(* Logix 5000 Rung export; software revision 16.04 *)

MODULES
   Local : vendor None type None code None
   EGD : vendor None type None code None
END_MODULES

TYPE SNTPStat :   // Simple Network Time Protocol statistics.
STRUCT
   ValidTime : INT;   // SNTP valid time
   ReqCnt : INT;   // SNTP request count
   RespCnt : INT;   // SNTP response count
   CompCnt : INT;   // SNTP computation count
   SetCnt : INT;   // SNTP set count
   TimeoutErrCnt : INT;   // SNTP timeout error count
   SecLSW : INT;   // SNTP seconds (LSW)
   SecMSW : INT;   // SNTP seconds (MSW)
   micSecLSW : INT;   // SNTP microseconds (LSW)
   micSecMSW : INT;   // SNTP microseconds (MSW)
   Sec : DINT;   // SNTP seconds
   micSec : DINT;   // SNTP microseconds
END_STRUCT
END_TYPE

TYPE InStat :   // This status data is returned on each read block and can be used to detect proper module operation.
STRUCT
   PassCnt : INT;   // Program cycle/scan counter
   BlkCntr : BlkStat;   // Block counter statistics
   SNTP : SNTPStat;   // Simple Network Time Protocol statistics
END_STRUCT
END_TYPE

TYPE EGDCONTROL :   // Stores control registers used by the processor to request special tasks from the module.
STRUCT
   ColdBoot : BOOL;   // Total SW/HW module reset
   WarmBoot : BOOL;   // Configuration parameter reset
   CPmessage : CPStat[17];   // CP message status
   CPmessReq : BOOL;   // Initiates Block 2000. C/P Messages
   CPmessReqQty : INT;   // Quantity of Consumer/Producer Message
   CPindxFirst : INT;   // Index of the First Consumer/Producer Message
   CPmessResQty : INT;   // Quantity of Consumer/Producer Message from Module
   CPindxResFirst : INT;   // Index of the First Consumer/Producer Message from Module
   CPwordsQty : INT;   // Calculated words Qty CP messages x 14.
   PortErrors : PortErrors;   // This encapsulates all port error statistics.
END_STRUCT
END_TYPE

TYPE BlkStat :   // Block Transfer Statistics
STRUCT
   Write : INT;   // Total number of write block transfers. Block Write counter.
   Read : INT;   // Total number of read block transfers. Block Read counter.
   Parse : INT;   // Total number of blocks parsed. Block Parse counter.
   Error : INT;   // Total number of block transfer errors. Block Error Counter.
END_STRUCT
END_TYPE

TYPE EGDMODULEDEF :   // MVI56-EGD module definitions.
STRUCT
   DATA : EGDDATA;   // Stores the database (read and write) values.
   CONTROL : EGDCONTROL;   // Stores control registers used by the processor to request special tasks from the module.
   STATUS : EGDSTATUS;   // Stores status registers.
   UTIL : EGDUTIL;   // Stores tags that are used by the ladder logic for internal processing.
END_STRUCT
END_TYPE

TYPE Blk9250Stat :   // Block 9250 Response Block general status
STRUCT
   BlkWriteIDreq : INT;   // Block Write ID Requested
   PassCnt : INT;   // Program Scan Counter
   ProdCodeByte0 : SINT;   // Product code byte 0 of 0 & 1
   ProdCodeByte1 : SINT;   // Product code byte 1 of 0 & 1
   ProdCodeByte2 : SINT;   // Product code byte 2 of 2 & 3
   ProdCodeByte3 : SINT;   // Product code byte 3 of 2 & 3
   RevByte0 : SINT;   // Revision byte 0 of 0 & 1
   RevByte1 : SINT;   // Revision byte 1 of 0 & 1
   RevByte2 : SINT;   // Revision byte 2 of 2 & 3
   RevByte3 : SINT;   // Revision byte 3 of 2 & 3
   OpByte0 : SINT;   // Op byte 0 of 0 & 1
   OpByte1 : SINT;   // Op byte 1 of 0 & 1
   OpByte2 : SINT;   // Op byte 2 of 2 & 3
   OpByte3 : SINT;   // Op byte 3 of 2 & 3
   RunByte0 : SINT;   // Run byte 0 of 0 & 1
   RunByte1 : SINT;   // Run byte 1 of 0 & 1
   RunByte2 : SINT;   // Run byte 2 of 2 & 3
   RunByte3 : SINT;   // Run byte 3 of 2 & 3
   BlkXferStat : BlkStat;   // Block transfer statistics
   ProductCodeName : DINT;   // Product code name
   RevisionLevel : DINT;   // Firmware revision level
   OpSysRevision : DINT;   // Operating system revision level
   RunNumber : DINT;   // Run number
END_STRUCT
END_TYPE

TYPE CPStat :   // Block 2000 Each Conmsumer/Producer Status Data
STRUCT
   Status : INT;   // Status (0=invalid, 1=producing/healthy, 2=pending/unhealthy)
   StatBit : INT;   // Status bit mapped (bit 0=error or invalid, bit 1=not time synchronized, bits 2 to 15 reserved)
   CPnumTimesLSW : INT;   // Number of times C/P (LSW)
   CPnumTimesMSW : INT;   // Number of times C/P (MSW)
   MissCntLSW : INT;   // Missed count (LSW)
   MissCntMSW : INT;   // Missed count (MSW)
   RfrshCntErrLSW : INT;   // Refresh count error (LSW)
   RfrshCntErrMSW : INT;   // Refresh count error (MSW)
   InvErrBit : INT;   // Invalid error bit set by producer
   TimeSyncErr : INT;   // Time sync error set by producer
   ShrtMEsgErr : INT;   // Short message error in exchange
   LngMEsgErr : INT;   // Long message error in exchange
   PrtclPVN : INT;   // Protocol PVN not set to 1
   CnfgSig : INT;   // Configuration signature not set correctly
   CPMessageCount : DINT;   // Number of times C/P
   MissedCount : DINT;   // Missed count
   RefreshCountErr : DINT;   // Refresh count error
END_STRUCT
END_TYPE

TYPE EGDUTIL :   // Stores tags that are used by the ladder logic for internal processing.
STRUCT
   HaltBlk9250 : BOOL;   // Halts Block 9250
   HaltBlk2000 : BOOL;   // Halts Block 2000
   BP : Backplane;   // Values used by program for data transfer operation between the module and the processor.
END_STRUCT
END_TYPE

TYPE EGDDATA :   // Stores the database (read and write) values.
STRUCT
   ReadData : INT[600];   // Data read from module
   WriteData : INT[600];   // Data to write to module
END_STRUCT
END_TYPE

TYPE EGDSTATUS :   // Stores status registers.
STRUCT
   Blk9250GenStat : Blk9250Stat;   // Block 9250 statistics
   BlkStat : BlkStat;   // Block Transfer Statistics
   CPStat : CPStat;   // Block 2000 Each Conmsumer/Producer Status Data
   InStat : InStat;   // Status information in each read block
   SNTPStat : SNTPStat;   // Simple Network Time Protocol statistics.
   GenStatReq : BOOL;   // Initiates Block 9260 C/P Messages
END_STRUCT
END_TYPE

TYPE Backplane :   // Values used by program for data transfer operation between the module and the processor.
STRUCT
   LastRead : INT;   // Index of last read block
   LastWrite : INT;   // Index of last write block
   BlockIndex : INT;   // Computed block offset for data table
   StatusIndex : INT;   // Computed block offset for status data
   ReadDataBlkCount : INT;   // Holds the value of the Block Counts of the Read Data Array. Array Size is divided by 200.
   WriteDataBlkCount : INT;   // Holds the value of the Block Counts of the Write Data Array. Array Size is divided by 200.
   RBTSremainder : INT;   // Holds remainder calculation value from the read array.
   WBTSremainder : INT;   // Holds remainder calculation value from the write array.
   ReadDataSizeGet : INT;   // Holds read data array size.
   WriteDataSizeGet : INT;   // Holds write data array size.
END_STRUCT
END_TYPE

TYPE PortErrors :   // This encapsulates all port error statistics.
STRUCT
   CmdReq : INT;   // Total number of command list requests sent
   CmdResp : INT;   // Total number of command list responses received
   CmdErr : INT;   // Total number of command list errors
   Requests : INT;   // Total number of requests for port
   Responses : INT;   // Total number of responses for port
   ErrSent : INT;   // Total number of errors sent
   ErrRec : INT;   // Total number of errors received
   CfgErrWord : INT;   // Configuration Error Word
   CurErr : INT;   // Current Error code
   LastErr : INT;   // Last recorded error code
END_STRUCT
END_TYPE

ADD_ON_INSTRUCTION AOI56EGD   (* revision 1.2, vendor ProSoft Technology, ExecutePrescan *)
// Add-On instruction for the MVI56-EGD module.
// Revision note:
// v1.2 - Removed FLL instruction in PreScan that was clearing WriteData Array in RUN/PROGRAM mode change
VAR_IN_OUT
   Connection_Input : INT[250]; {required}   // Input parameters.
   Connection_Output : INT[248]; {required}   // Output parameters
   EGD : EGDMODULEDEF; {required}
END_VAR
VAR
   MJFaults : DINT[12];
END_VAR

ROUTINE Logic   (* ladder *)
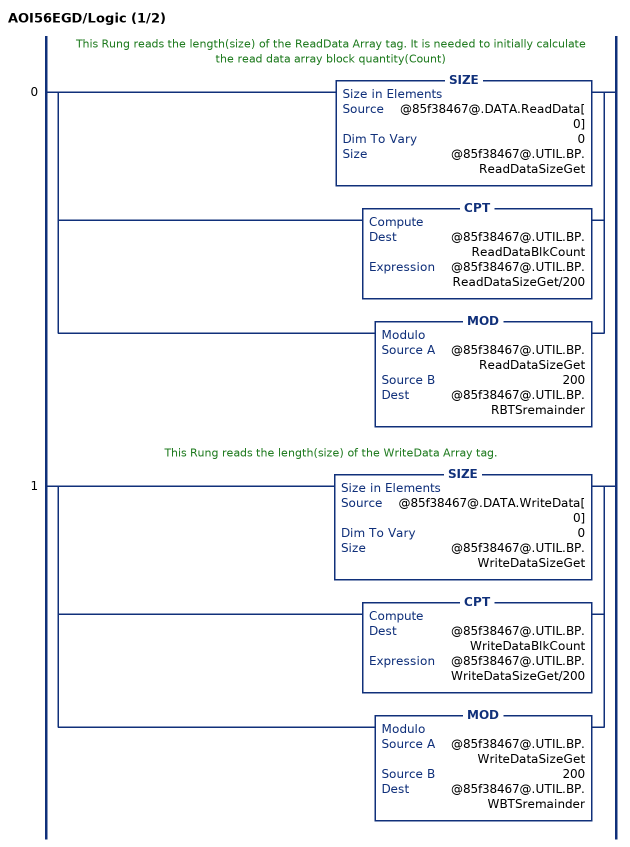
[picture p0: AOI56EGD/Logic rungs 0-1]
   // This Rung reads the length(size) of the ReadData Array tag. It is needed to initially calculate the read data array block quantity(Count)
   0: [SIZE(@85f38467@.DATA.ReadData[0],0,@85f38467@.UTIL.BP.ReadDataSizeGet) ,CPT(@85f38467@.UTIL.BP.ReadDataBlkCount,@85f38467@.UTIL.BP.ReadDataSizeGet/200) ,MOD(@85f38467@.UTIL.BP.ReadDataSizeGet,200,@85f38467@.UTIL.BP.RBTSremainder) ];
   // This Rung reads the length(size) of the WriteData Array tag.
   1: [SIZE(@85f38467@.DATA.WriteData[0],0,@85f38467@.UTIL.BP.WriteDataSizeGet) ,CPT(@85f38467@.UTIL.BP.WriteDataBlkCount,@85f38467@.UTIL.BP.WriteDataSizeGet/200) ,MOD(@85f38467@.UTIL.BP.WriteDataSizeGet,200,@85f38467@.UTIL.BP.WBTSremainder) ];
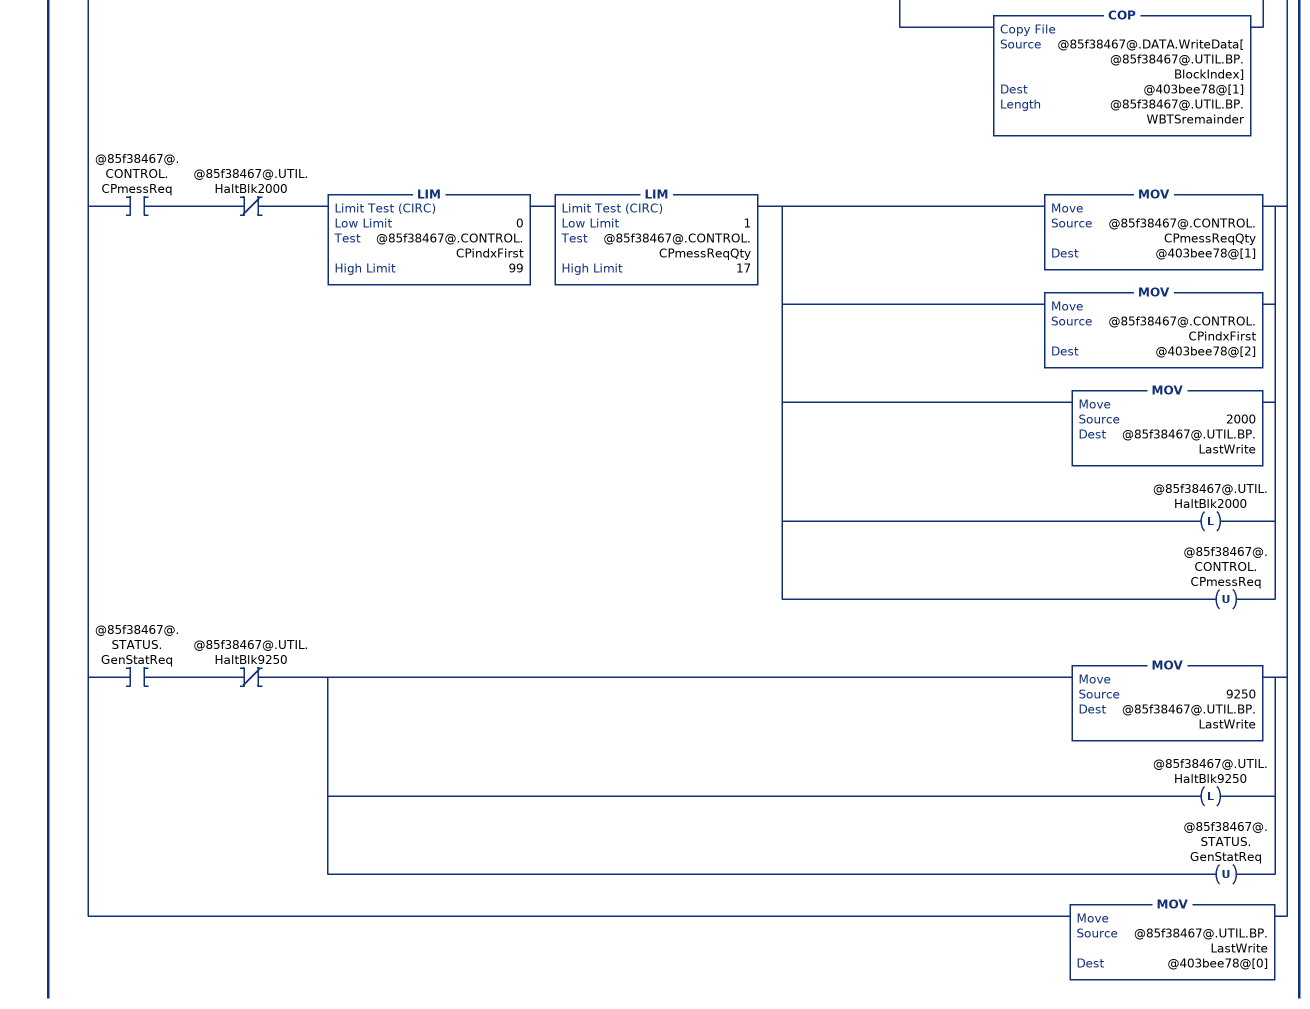
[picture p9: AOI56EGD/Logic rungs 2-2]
   2: NEQ(@65a9e839@[249],@85f38467@.UTIL.BP.LastRead)[MOV(@65a9e839@[249],@85f38467@.UTIL.BP.LastRead) ,GEQ(@85f38467@.UTIL.BP.LastRead,1) [LEQ(@85f38467@.UTIL.BP.LastRead,@85f38467@.UTIL.BP.ReadDataBlkCount) [CPT(@85f38467@.UTIL.BP.BlockIndex,(@85f38467@.UTIL.BP.LastRead-1)*200) ,COP(@65a9e839@[2],@85f38467@.DATA.ReadData[@85f38467@.UTIL.BP.BlockIndex],200) ] ,CMP(@85f38467@.UTIL.BP.LastRead - @85f38467@.UTIL.BP.ReadDataBlkCount = 1) GRT(@85f38467@.UTIL.BP.RBTSremainder,0) [CPT(@85f38467@.UTIL.BP.BlockIndex,(@85f38467@.UTIL.BP.LastRead-1) * 200) ,COP(@65a9e839@[2],@85f38467@.DATA.ReadData[@85f38467@.UTIL.BP.BlockIndex],@85f38467@.UTIL.BP.RBTSremainder) ] ] ,[COP(@65a9e839@[202],@85f38467@.STATUS.InStat.PassCnt,1) ,COP(@65a9e839@[203],@85f38467@.STATUS.InStat.BlkCntr.Write,4) ,COP(@65a9e839@[207],@85f38467@.STATUS.InStat.SNTP.ValidTime,10) ,COP(@85f38467@.STATUS.InStat.SNTP.SecLSW,@85f38467@.STATUS.InStat.SNTP.Sec,2) ] ,EQU(@85f38467@.UTIL.BP.LastRead,2000) [MOV(@65a9e839@[2],@85f38467@.CONTROL.CPmessResQty) ,MOV(@65a9e839@[3],@85f38467@.CONTROL.CPindxResFirst) ,[COP(@65a9e839@[4],@85f38467@.CONTROL.CPmessage[0].Status,14) ,COP(@85f38467@.CONTROL.CPmessage[0].CPnumTimesLSW,@85f38467@.CONTROL.CPmessage[0].CPMessageCount,3) ] ,[COP(@65a9e839@[18],@85f38467@.CONTROL.CPmessage[1].Status,14) ,COP(@85f38467@.CONTROL.CPmessage[1].CPnumTimesLSW,@85f38467@.CONTROL.CPmessage[1].CPMessageCount,3) ] ,[COP(@65a9e839@[32],@85f38467@.CONTROL.CPmessage[2].Status,14) ,COP(@85f38467@.CONTROL.CPmessage[2].CPnumTimesLSW,@85f38467@.CONTROL.CPmessage[2].CPMessageCount,3) ] ,[COP(@65a9e839@[46],@85f38467@.CONTROL.CPmessage[3].Status,14) ,COP(@85f38467@.CONTROL.CPmessage[3].CPnumTimesLSW,@85f38467@.CONTROL.CPmessage[3].CPMessageCount,3) ] ,[COP(@65a9e839@[60],@85f38467@.CONTROL.CPmessage[4].Status,14) ,COP(@85f38467@.CONTROL.CPmessage[4].CPnumTimesLSW,@85f38467@.CONTROL.CPmessage[4].CPMessageCount,3) ] ,[COP(@65a9e839@[74],@85f38467@.CONTROL.CPmessage[5].Status,14) ,COP(@85f38467@.CONTROL.CPmessage[5].CPnumTimesLSW,@85f38467@.CONTROL.CPmessage[5].CPMessageCount,3) ] ,[COP(@65a9e839@[88],@85f38467@.CONTROL.CPmessage[6].Status,14) ,COP(@85f38467@.CONTROL.CPmessage[6].CPnumTimesLSW,@85f38467@.CONTROL.CPmessage[6].CPMessageCount,3) ] ,[COP(@65a9e839@[102],@85f38467@.CONTROL.CPmessage[7].Status,14) ,COP(@85f38467@.CONTROL.CPmessage[7].CPnumTimesLSW,@85f38467@.CONTROL.CPmessage[7].CPMessageCount,3) ] ,[COP(@65a9e839@[116],@85f38467@.CONTROL.CPmessage[8].Status,14) ,COP(@85f38467@.CONTROL.CPmessage[8].CPnumTimesLSW,@85f38467@.CONTROL.CPmessage[8].CPMessageCount,3) ] ,[COP(@65a9e839@[130],@85f38467@.CONTROL.CPmessage[9].Status,14) ,COP(@85f38467@.CONTROL.CPmessage[9].CPnumTimesLSW,@85f38467@.CONTROL.CPmessage[9].CPMessageCount,3) ] ,[COP(@65a9e839@[144],@85f38467@.CONTROL.CPmessage[10].Status,14) ,COP(@85f38467@.CONTROL.CPmessage[10].CPnumTimesLSW,@85f38467@.CONTROL.CPmessage[10].CPMessageCount,3) ] ,[COP(@65a9e839@[158],@85f38467@.CONTROL.CPmessage[11].Status,14) ,COP(@85f38467@.CONTROL.CPmessage[11].CPnumTimesLSW,@85f38467@.CONTROL.CPmessage[11].CPMessageCount,3) ] ,[COP(@65a9e839@[172],@85f38467@.CONTROL.CPmessage[12].Status,14) ,COP(@85f38467@.CONTROL.CPmessage[12].CPnumTimesLSW,@85f38467@.CONTROL.CPmessage[12].CPMessageCount,3) ] ,[COP(@65a9e839@[186],@85f38467@.CONTROL.CPmessage[13].Status,14) ,COP(@85f38467@.CONTROL.CPmessage[13].CPnumTimesLSW,@85f38467@.CONTROL.CPmessage[13].CPMessageCount,3) ] ,[COP(@65a9e839@[200],@85f38467@.CONTROL.CPmessage[14].Status,14) ,COP(@85f38467@.CONTROL.CPmessage[14].CPnumTimesLSW,@85f38467@.CONTROL.CPmessage[14].CPMessageCount,3) ] ,[COP(@65a9e839@[214],@85f38467@.CONTROL.CPmessage[15].Status,14) ,COP(@85f38467@.CONTROL.CPmessage[15].CPnumTimesLSW,@85f38467@.CONTROL.CPmessage[15].CPMessageCount,3) ] ,[COP(@65a9e839@[228],@85f38467@.CONTROL.CPmessage[16].Status,14) ,COP(@85f38467@.CONTROL.CPmessage[16].CPnumTimesLSW,@85f38467@.CONTROL.CPmessage[16].CPMessageCount,3) ] ,OTU(@85f38467@.UTIL.HaltBlk2000) ] ,EQU(@85f38467@.UTIL.BP.LastRead,9250) [MOV(@65a9e839@[1],@85f38467@.STATUS.Blk9250GenStat.BlkWriteIDreq) ,COP(@65a9e839@[2],@85f38467@.STATUS.Blk9250GenStat.PassCnt,1) ,[COP(@65a9e839@[3],@85f38467@.STATUS.Blk9250GenStat.ProdCodeByte0,16) ,COP(@85f38467@.STATUS.Blk9250GenStat.ProdCodeByte0,@85f38467@.STATUS.Blk9250GenStat.ProductCodeName,4) ,SWPB(@85f38467@.STATUS.Blk9250GenStat.ProductCodeName,REVERSE,@85f38467@.STATUS.Blk9250GenStat.ProductCodeName) ,SWPB(@85f38467@.STATUS.Blk9250GenStat.RevisionLevel,REVERSE,@85f38467@.STATUS.Blk9250GenStat.RevisionLevel) ,SWPB(@85f38467@.STATUS.Blk9250GenStat.OpSysRevision,REVERSE,@85f38467@.STATUS.Blk9250GenStat.OpSysRevision) ,SWPB(@85f38467@.STATUS.Blk9250GenStat.RunNumber,REVERSE,@85f38467@.STATUS.Blk9250GenStat.RunNumber) ] ,COP(@65a9e839@[11],@85f38467@.STATUS.Blk9250GenStat.BlkXferStat.Write,4) ,[COP(@65a9e839@[15],@85f38467@.STATUS.SNTPStat.ValidTime,10) ,COP(@85f38467@.STATUS.SNTPStat.SecLSW,@85f38467@.STATUS.SNTPStat.Sec,2) ] ,OTU(@85f38467@.UTIL.HaltBlk9250) ] ,MOV(@65a9e839@[1],@85f38467@.UTIL.BP.LastWrite) ,XIC(@85f38467@.CONTROL.WarmBoot) [MOV(9998,@85f38467@.UTIL.BP.LastWrite) ,OTU(@85f38467@.CONTROL.WarmBoot) ] ,XIC(@85f38467@.CONTROL.ColdBoot) [MOV(9999,@85f38467@.UTIL.BP.LastWrite) ,OTU(@85f38467@.CONTROL.ColdBoot) ] ,GEQ(@85f38467@.UTIL.BP.LastWrite,1) [LEQ(@85f38467@.UTIL.BP.LastWrite,@85f38467@.UTIL.BP.WriteDataBlkCount) [CPT(@85f38467@.UTIL.BP.BlockIndex,(@85f38467@.UTIL.BP.LastWrite-1)*200) ,COP(@85f38467@.DATA.WriteData[@85f38467@.UTIL.BP.BlockIndex],@403bee78@[1],200) ] ,CMP(@85f38467@.UTIL.BP.LastWrite - @85f38467@.UTIL.BP.WriteDataBlkCount = 1) GRT(@85f38467@.UTIL.BP.WBTSremainder,0) [CPT(@85f38467@.UTIL.BP.BlockIndex,(@85f38467@.UTIL.BP.LastWrite-1)*200) ,COP(@85f38467@.DATA.WriteData[@85f38467@.UTIL.BP.BlockIndex],@403bee78@[1],@85f38467@.UTIL.BP.WBTSremainder) ] ] ,XIC(@85f38467@.CONTROL.CPmessReq) XIO(@85f38467@.UTIL.HaltBlk2000) LIM(0,@85f38467@.CONTROL.CPindxFirst,99) LIM(1,@85f38467@.CONTROL.CPmessReqQty,17) [MOV(@85f38467@.CONTROL.CPmessReqQty,@403bee78@[1]) ,MOV(@85f38467@.CONTROL.CPindxFirst,@403bee78@[2]) ,MOV(2000,@85f38467@.UTIL.BP.LastWrite) ,OTL(@85f38467@.UTIL.HaltBlk2000) ,OTU(@85f38467@.CONTROL.CPmessReq) ] ,XIC(@85f38467@.STATUS.GenStatReq) XIO(@85f38467@.UTIL.HaltBlk9250) [MOV(9250,@85f38467@.UTIL.BP.LastWrite) ,OTL(@85f38467@.UTIL.HaltBlk9250) ,OTU(@85f38467@.STATUS.GenStatReq) ] ,MOV(@85f38467@.UTIL.BP.LastWrite,@403bee78@[0]) ];
END_ROUTINE

ROUTINE Prescan   (* ladder *)
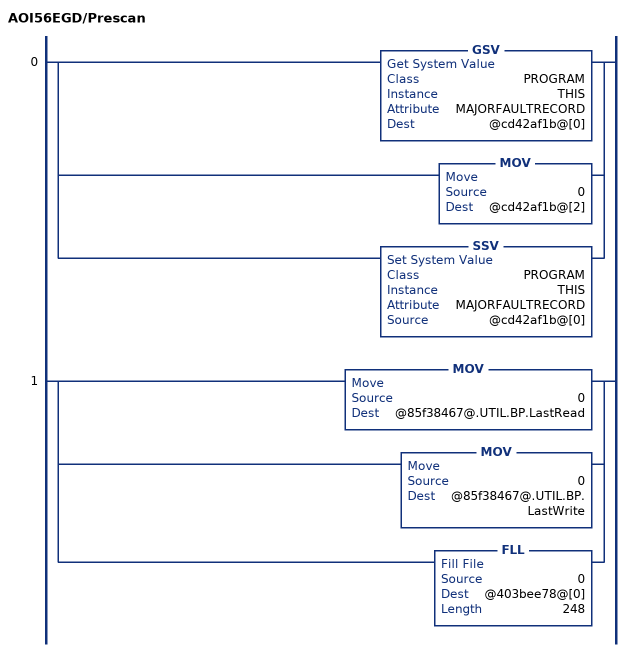
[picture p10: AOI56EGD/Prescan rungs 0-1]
   0: [GSV(PROGRAM,THIS,MAJORFAULTRECORD,@cd42af1b@[0]) ,MOV(0,@cd42af1b@[2]) ,SSV(PROGRAM,THIS,MAJORFAULTRECORD,@cd42af1b@[0]) ];
   1: [MOV(0,@85f38467@.UTIL.BP.LastRead) ,MOV(0,@85f38467@.UTIL.BP.LastWrite) ,FLL(0,@403bee78@[0],248) ];
END_ROUTINE
END_ADD_ON_INSTRUCTION

VAR_GLOBAL   (* controller tags *)
   AOI56EGD : AOI56EGD;
   Local:1:O : AB:1756_MODULE_INT_496Bytes:O:0;
   EGD : EGDMODULEDEF;
   Local:1:I : AB:1756_MODULE_INT_500Bytes:I:0;
END_VAR

PROGRAM MainProgram

ROUTINE MainRoutine   (* ladder *)
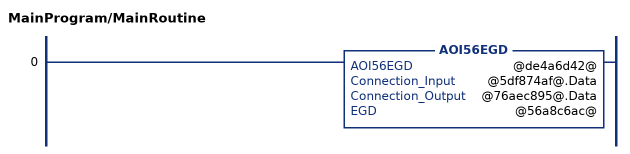
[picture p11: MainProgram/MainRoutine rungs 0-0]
   0: AOI56EGD(@de4a6d42@,@5df874af@.Data,@76aec895@.Data,@56a8c6ac@);
END_ROUTINE
END_PROGRAM
